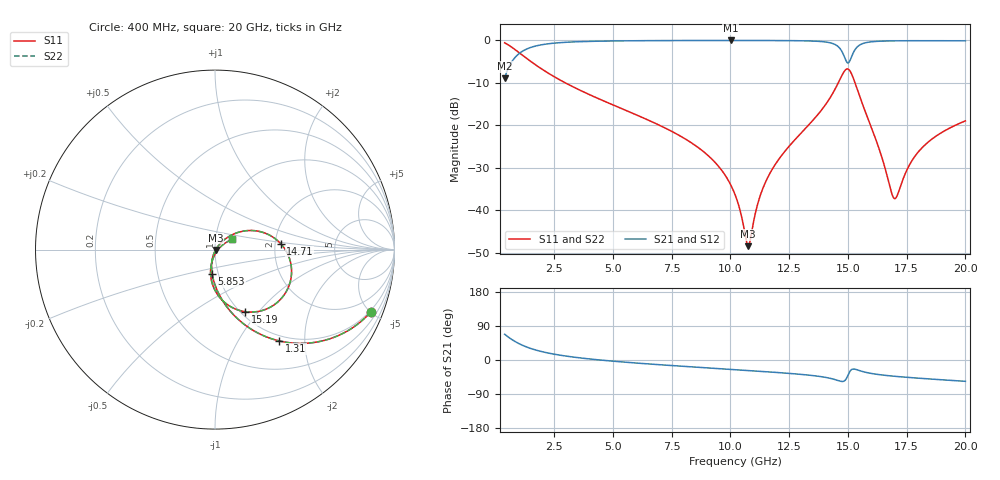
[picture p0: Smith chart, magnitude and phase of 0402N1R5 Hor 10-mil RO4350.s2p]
# GHz S MA R 50
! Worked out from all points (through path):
!   1960 points, 400 MHz to 20 GHz, reference 50 ohm
!   highest |S21| = -0.03 dB at 10.02 GHz (marker M1); lowest = -9.0 dB at 400 MHz (marker M2)
!   group delay of S21, straight-line fit = 12.2 ps
!   lowest |S11| = -48.4 dB at 10.77 GHz (marker M3), VSWR 1.01, Z = 50.3 - j0.178 ohm
!   |S11| at or under -10 dB: 2.978 GHz to 14.59 GHz (11.62 GHz wide, 132 % of centre); 15.3 GHz to end of sweep
!   |S22| runs from -48.4 to -0.6 dB; largest |S21 - S12| = 0
!   S11 on the Smith chart (normalised r, x): 400 MHz: 0.91, -5.00; 1.31 GHz: 0.91, -1.51; 5.853 GHz: 0.93, -0.26; 14.71 GHz: 2.14, +0.17; 15.19 GHz: 1.05, -0.86; 20 GHz: 1.21, +0.14
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0.4  0.9342 -21.9  0.3565 68.0  0.3565 68.0  0.9342 -21.9
0.8102093  0.79 -39.9  0.6125 50.1  0.6125 50.1  0.79 -39.9
1.310465  0.6207 -55.0  0.7832 34.9  0.7832 34.9  0.6207 -55.0
2.230934  0.4149 -71.2  0.9086 18.7  0.9086 18.7  0.4149 -71.2
3.671669  0.2536 -84.5  0.9655 5.1  0.9655 5.1  0.2536 -84.5
5.852782  0.1382 -96.4  0.9879 -7.3  0.9879 -7.3  0.1382 -96.4
6.943338  0.1014 -100.9  0.9921 -12.3  0.9921 -12.3  0.1014 -100.9
8.914344  0.04763 -106.8  0.9955 -20.4  0.9955 -20.4  0.04763 -106.8
10.02491  0.01973 -105.0  0.996 -24.8  0.996 -24.8  0.01973 -105.0
10.205  0.01521 -102.4  0.996 -25.5  0.996 -25.5  0.01521 -102.4
10.76529  0.003783 -27.9  0.9958 -27.8  0.9958 -27.8  0.003783 -27.9
11.21552  0.01326 42.2  0.9953 -29.6  0.9953 -29.6  0.01326 42.2
11.63573  0.02568 48.3  0.9946 -31.4  0.9946 -31.4  0.02568 48.3
13.46667  0.1107 42.7  0.9808 -40.8  0.9808 -40.8  0.1107 42.7
14.7073  0.3669 5.3  0.7713 -56.3  0.7713 -56.3  0.3669 5.3
14.93742  0.4574 -24.5  0.5648 -48.9  0.5648 -48.9  0.4574 -24.5
15.18754  0.3856 -63.9  0.6713 -24.4  0.6713 -24.4  0.3856 -63.9
15.58775  0.1886 -94.8  0.9051 -29.7  0.9051 -29.7  0.1886 -94.8
16.73834  0.02145 -83.1  0.9832 -41.5  0.9832 -41.5  0.02145 -83.1
17.02848  0.01384 -27.5  0.986 -43.2  0.986 -43.2  0.01384 -27.5
18.08903  0.05197 31.7  0.989 -48.4  0.989 -48.4  0.05197 31.7
20  0.1127 30.2  0.9859 -56.3  0.9859 -56.3  0.1127 30.2
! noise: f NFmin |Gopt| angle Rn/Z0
0.4  0.001296  0.8073  4.832  0.001397
2.571  0.005059  0.6796  8.449  0.003038
4.752  0.008058  0.6378  13.55  0.00414
6.933  0.01083  0.615  18.77  0.005101
9.104  0.01372  0.6067  23.92  0.006194
11.29  0.01784  0.6254  28.98  0.008385
13.47  0.03317  0.7457  34.17  0.024
15.64  0.0859  0.8793  39.76  0.1362
17.82  0.03289  0.6841  44.63  0.01738
20  0.02968  0.6279  49.07  0.01251
